[IBIS Ver]   4.2
[File Name]  stm32f2_lqfp144.ibs
[File Rev]   1.0
[Date]   31-Aug-2011
[Source]   STMicroelectronics NV
[Notes]   The I/O models have been made by simulation and qualified
   with recomandation of QualityIBIS flow.
   Some Models, library and pin names may be modified.
   Details of modified names can be found below.
ORIGINAL NAME   ::  MODIFIED NAME   :: COMMENTS(if any)
IO8USB_LSFS_OTG_FT  ::  IO8USB_LSFS_OTG_FT_USB   :: Model in USB mode.
IO8USB_LSFS_OTG_FT  ::  IO8USB_LSFS_OTG_FT_NON_USB_DNV33  :: Model in other than USB mode & pad pin = DNV33
IO8USB_LSFS_OTG_FT  ::  IO8USB_LSFS_OTG_FT_NON_USB_DPV33  :: Model in other than USB mode & pad pin = DPV33
[Disclaimer] These IBIS models are the proprietary information of
   STMicroelectronics and are disclosed to users solely for
   modeling and simulation purposes. No further license is
   implied. All warranties express, implied, or statutory,
   including any implied warranty of fitness for a particular
   purpose or implied warranty against infringement, are
   hereby disclaimed. STMicroelectronics reserves the right
   to change the IBIS models at any time and without notice.
[Copyright]  (c) STMicroelectronics
   All rights reserved. Reproduction in whole or part is prohibited
   without the written consent of the copyright holder.
[Component]  STM32F2_LQFP144
[Manufacturer] STMicroelectronics NV
[Package]
| variable   typ   min   max
R_pkg   0.000mOhm   0.000mOhm   0.000mOhm
L_pkg   0.000nH   0.000nH   0.000nH
C_pkg   0.000pF   0.000pF   0.000pF
[Pin]   signal_name   model_name
1 PE2 IO8PROG2M25M50M100M_ARSUDQ_FT
2 PE3 IO8PROG2M25M50M100M_ARSUDQ_FT
3 PE4 IO8PROG2M25M50M100M_ARSUDQ_FT
4 PE5 IO8PROG2M25M50M100M_ARSUDQ_FT
5 PE6 IO8PROG2M25M50M100M_ARSUDQ_FT
|6 VBAT VDD33IOSWCO_MOSSWI_FT
|- PI8 IO8PROG2M25M50M100M_ARSUDQ_FT_V33
7 PC13 IO8PROG2M25M50M100M_ARWSUDQ_FT_V33
8 PC14 IO8PROG2M25M50M100M_ARWSUDQ_FT
9 PC15 IO8PROG2M25M50M100M_ARSUDQ_FT
|- PI9  IO8PROG2M25M50M100M_ARSUDQ_FT
|- PI10 IO8PROG2M25M50M100M_ARSUDQ_FT
|- PI11 IO8PROG2M25M50M100M_ARSUDQ_FT
|- VSS_13 VSSIOCO
|- VDD_13 VDD33IOCO
10 PF0 IO8PROG2M25M50M100M_ARSUDQ_FT
11 PF1 IO8PROG2M25M50M100M_ARSUDQ_FT
12 PF2 IO8PROG2M25M50M100M_ARSUDQ_FT
13 PF3 IO8PROG2M25M50M100M_ARSUDQ_FT
14 PF4 IO8PROG2M25M50M100M_ARSUDQ_FT
15 PF5 IO8PROG2M25M50M100M_ARSUDQ_FT
|16 VSS_5 VSSIOCO
|17 VDD_5 VDD33IOCO
18 PF6 IO8PROG2M25M50M100M_ARSUDQ_FT
19 PF7 IO8PROG2M25M50M100M_ARSUDQ_FT
20 PF8 IO8PROG2M25M50M100M_ARSUDQ_FT
21 PF9  IO8PROG2M25M50M100M_AR3WSUDQ_FT
22 PF10 IO8PROG2M25M50M100M_ARSUDQ_FT
23 PH0 IO8PROG2M25M50M100M_ARSUDQ_FT
24 PH1 IO8PROG2M25M50M100M_ARSUDQ_FT
|25 NRST RESET
26 PC0 IO8PROG2M25M50M100M_AR3WSUDQ_FT
27 PC1 IO8PROG2M25M50M100M_AR3WSUDQ_FT
28 PC2 IO8PROG2M25M50M100M_AR3WSUDQ_FT
29 PC3 IO8PROG2M25M50M100M_AR3WSUDQ_FT
|30 VDD_12 VDD33IOCO_VSSIOCO_MOSSWI_FT
|31 VSSA VSSCO
|32 VREF+ VDD33CO
|33 VDDA VDD33CO
34 PA0 IO8PROG2M25M50M100M_AR3WSUDQ_FT_V33
35 PA1 IO8PROG2M25M50M100M_AR3WSUDQ_FT
36 PA2 IO8PROG2M25M50M100M_AR3WSUDQ_FT
|- PH2 IO8PROG2M25M50M100M_AR3WSUDQ_FT
|- PH3 IO8PROG2M25M50M100M_AR3WSUDQ_FT
|- PH4 IO8PROG2M25M50M100M_AR3WSUDQ_FT
|- PH5 IO8PROG2M25M50M100M_AR3WSUDQ_FT
37 PA3 IO8PROG2M25M50M100M_AR3WSUDQ_FT
|38 VSS_4 VSSIOCO
|39 VDD_4 VDD33IOCO
40 PA4 IO8PROG2M25M50M100M_AR3WSUDQ_FT
41 PA5 IO8PROG2M25M50M100M_AR3WSUDQ_FT
42 PA6 IO8PROG2M25M50M100M_AR3WSUDQ_FT
43 PA7 IO8PROG2M25M50M100M_AR3WSUDQ_FT
44 PC4 IO8PROG2M25M50M100M_AR3WSUDQ_FT
45 PC5 IO8PROG2M25M50M100M_AR3WSUDQ_FT
46 PB0 IO8PROG2M25M50M100M_AR3WSUDQ_FT
47 PB1 IO8PROG2M25M50M100M_AR3WSUDQ_FT
48 PB2 IO8PROG2M25M50M100M_AR3WSUDQ_FT
49 PF11 IO8PROG2M25M50M100M_ARSUDQ_FT
50 PF12 IO8PROG2M25M50M100M_ARSUDQ_FT
|51 VSS_6 VSSIOCO
|52 VDD_6 VDD33IOCO
53 PF13 IO8PROG2M25M50M100M_ARSUDQ_FT
54 PF14 IO8PROG2M25M50M100M_ARSUDQ_FT
55 PF15 IO8PROG2M25M50M100M_ARSUDQ_FT
56 PG0 IO8PROG2M25M50M100M_ARSUDQ_FT
57 PG1 IO8PROG2M25M50M100M_ARSUDQ_FT
58 PE7 IO8PROG2M25M50M100M_ARSUDQ_FT
59 PE8 IO8PROG2M25M50M100M_ARSUDQ_FT
60 PE9 IO8PROG2M25M50M100M_ARSUDQ_FT
|61 VSS_7 VSSIOCO
|62 VDD_7 VDD33IOCO
63 PE10 IO8PROG2M25M50M100M_ARSUDQ_FT
64 PE11 IO8PROG2M25M50M100M_ARSUDQ_FT
65 PE12 IO8PROG2M25M50M100M_ARSUDQ_FT
66 PE13 IO8PROG2M25M50M100M_ARSUDQ_FT
67 PE14 IO8PROG2M25M50M100M_ARSUDQ_FT
68 PE15 IO8PROG2M25M50M100M_ARSUDQ_FT
69 PB10 IO8PROG2M25M50M100M_ARSUDQ_I2CIN_FT
70 PB11 IO8PROG2M25M50M100M_ARSUDQ_I2CIN_FT
|71 VCAP_1
|72 VDD_1 VDD33IOCO
|- PH6 IO8PROG2M25M50M100M_ARSUDQ_FT
|- PH7 IO8PROG2M25M50M100M_ARSUDQ_FT
|- PH8 IO8PROG2M25M50M100M_ARSUDQ_FT
|- PH9 IO8PROG2M25M50M100M_ARSUDQ_FT
|- PH10 IO8PROG2M25M50M100M_ARSUDQ_FT
|- PH11 IO8PROG2M25M50M100M_ARSUDQ_FT
|- PH12 IO8PROG2M25M50M100M_ARSUDQ_FT
|- VSS_14 VSSIOCO
|- VDD_14 VDD33IOCO
73 PB12 IO8USB_ID_OTG_FT
74 PB13 IO8USB_VBUS_OTG_FT
75 PB14 IO8USB_LSFS_OTG_FT_USB
|75 PB14 IO8USB_LSFS_OTG_FT_NON_USB_DNV33
76 PB15 IO8USB_LSFS_OTG_FT_USB
|76 PB15 IO8USB_LSFS_OTG_FT_NON_USB_DPV3394
77 PD8 IO8PROG2M25M50M100M_ARSUDQ_FT
78 PD9 IO8PROG2M25M50M100M_ARSUDQ_FT
79 PD10 IO8PROG2M25M50M100M_ARSUDQ_FT
80 PD11 IO8PROG2M25M50M100M_ARSUDQ_FT
81 PD12 IO8PROG2M25M50M100M_ARSUDQ_FT
82 PD13 IO8PROG2M25M50M100M_ARSUDQ_FT
|83 VSS_8 VSSIOCO
|84 VDD_8 VDD33IOCO
85 PD14 IO8PROG2M25M50M100M_ARSUDQ_FT
86 PD15 IO8PROG2M25M50M100M_ARSUDQ_FT
87 PG2 IO8PROG2M25M50M100M_ARSUDQ_FT
88 PG3 IO8PROG2M25M50M100M_ARSUDQ_FT
89 PG4 IO8PROG2M25M50M100M_ARSUDQ_FT
90 PG5 IO8PROG2M25M50M100M_ARSUDQ_FT
91 PG6 IO8PROG2M25M50M100M_ARSUDQ_FT
92 PG7 IO8PROG2M25M50M100M_ARSUDQ_FT
93 PG8 IO8PROG2M25M50M100M_ARSUDQ_FT
|94 VSS_9 VSSIOCO
|95 VDD_9 VDD33IOCO
96 PC6 IO8PROG2M25M50M100M_ARSUDQ_FT
97 PC7 IO8PROG2M25M50M100M_ARSUDQ_FT
98 PC8 IO8PROG2M25M50M100M_ARSUDQ_FT
99 PC9 IO8PROG2M25M50M100M_ARSUDQ_I2CIN_FT
100 PA8 IO8PROG2M25M50M100M_ARSUDQ_I2CIN_FT
101 PA9 IO8USB_VBUS_OTG_FT
102 PA10 IO8USB_ID_OTG_FT
|103 PA11 IO8USB_LSFS_OTG_FT_USB
103 PA11 IO8USB_LSFS_OTG_FT_NON_USB_DNV33
|104 PA12 IO8USB_LSFS_OTG_FT_USB
104 PA12 IO8USB_LSFS_OTG_FT_NON_USB_DPV33
105 PA13 IO8PROG2M25M50M100M_ARSUDQ_FT
|106 VCAP_2
|107 VSS_2 VSSIOCO
|108 VDD_2 VDD33IOCO
|- PH13 IO8PROG2M25M50M100M_ARSUDQ_FT
|- PH14 IO8PROG2M25M50M100M_ARSUDQ_FT
|- PH15 IO8PROG2M25M50M100M_ARSUDQ_FT
|- PI0 IO8PROG2M25M50M100M_ARSUDQ_FT
|- PI1 IO8PROG2M25M50M100M_ARSUDQ_FT
|- PI2 IO8PROG2M25M50M100M_ARSUDQ_FT
|- PI3 IO8PROG2M25M50M100M_ARSUDQ_FT
|- VSS_15 VSSIOCO
|- VDD_15 VDD33IOCO
109 PA14 IO8PROG2M25M50M100M_ARSUDQ_FT
110 PA15 IO8PROG2M25M50M100M_AR3WSUDQ_FT
111 PC10 IO8PROG2M25M50M100M_ARSUDQ_FT
112 PC11 IO8PROG2M25M50M100M_ARSUDQ_FT
113 PC12 IO8PROG2M25M50M100M_ARSUDQ_FT
114 PD0 IO8PROG2M25M50M100M_ARSUDQ_FT
115 PD1 IO8PROG2M25M50M100M_ARSUDQ_FT
116 PD2 IO8PROG2M25M50M100M_ARSUDQ_FT
117 PD3 IO8PROG2M25M50M100M_ARSUDQ_FT
118 PD4 IO8PROG2M25M50M100M_ARSUDQ_FT
119 PD5 IO8PROG2M25M50M100M_ARSUDQ_FT
|120 VSS_10 VSSIOCO
|121 VDD_10 VDD33IOCO
122 PD6 IO8PROG2M25M50M100M_ARSUDQ_FT
123 PD7 IO8PROG2M25M50M100M_ARSUDQ_FT
124 PG9 IO8PROG2M25M50M100M_ARSUDQ_FT
125 PG10 IO8PROG2M25M50M100M_ARSUDQ_FT
126 PG11 IO8PROG2M25M50M100M_ARSUDQ_FT
127 PG12 IO8PROG2M25M50M100M_ARSUDQ_FT
128 PG13 IO8PROG2M25M50M100M_ARSUDQ_FT
129 PG14 IO8PROG2M25M50M100M_ARSUDQ_FT
|130 VSS_11 VSSIOCO
|131 VDD_11 VDD33IOCO
132 PG15 IO8PROG2M25M50M100M_ARSUDQ_FT
133 PB3 IO8PROG2M25M50M100M_ARSUDQ_FT
134 PB4 IO8PROG2M25M50M100M_ARSUDQ_FT
135 PB5 IO8PROG2M25M50M100M_AR3WSUDQ_FT
136 PB6 IO8PROG2M25M50M100M_ARSUDQ_I2CIN_FT
137 PB7 IO8PROG2M25M50M100M_ARSUDQ_I2CIN_FT
138 BOOT0 VPP_TEST_HV
139 PB8 IO8PROG2M25M50M100M_ARSUDQ_I2CIN_FT
140 PB9 IO8PROG2M25M50M100M_ARSUDQ_I2CIN_FT
141 PE0 IO8PROG2M25M50M100M_ARSUDQ_FT
142 PE1 IO8PROG2M25M50M100M_ARSUDQ_FT
|- VSS VSSIOCO
|143 RFU VSSIOCO
|144 VDD_3 VDD33IOCO
|- PI4 IO8PROG2M25M50M100M_ARSUDQ_FT
|- PI5 IO8PROG2M25M50M100M_ARSUDQ_FT
|- PI6 IO8PROG2M25M50M100M_ARSUDQ_FT
|- PI7 IO8PROG2M25M50M100M_ARSUDQ_FT
[Diff Pin]  inv_pin   vdiff tdelay_typ tdelay_min tdelay_max
75 76 200mV 0  0 0
103 104 200mV 0  0 0
[Model Selector] IO8PROG2M25M50M100M_AR3WSUDQ_FT_V33
IO8PROG2M25M50M100M_AR3WSUDQ_DRV_V33_00   DRIVER MODEL  : SPEEDAV33=0 SPEEDBV33=0
IO8PROG2M25M50M100M_AR3WSUDQ_DRV_V33_01   DRIVER MODEL  : SPEEDAV33=0 SPEEDBV33=1
IO8PROG2M25M50M100M_AR3WSUDQ_DRV_V33_10   DRIVER MODEL  : SPEEDAV33=1 SPEEDBV33=0
IO8PROG2M25M50M100M_AR3WSUDQ_DRV_V33_11   DRIVER MODEL  : SPEEDAV33=1 SPEEDBV33=1
IO8PROG2M25M50M100M_AR3WSUDQ_RCV_V33_0   CMOS RECIEVER : ENHYSV33=0  OUTPUT=ZIV33
IO8PROG2M25M50M100M_AR3WSUDQ_RCV_V33_0_T  TTL  RECIEVER : ENHYSV33=0  OUTPUT=ZIV33
IO8PROG2M25M50M100M_AR3WSUDQ_RCV_V33_1   CMOS RECIEVER : ENHYSV33=1  OUTPUT=ZIV33
IO8PROG2M25M50M100M_AR3WSUDQ_RCV_V33_1_T  TTL  RECIEVER : ENHYSV33=1  OUTPUT=ZIV33
[Model Selector] IO8PROG2M25M50M100M_AR3WSUDQ_FT
IO8PROG2M25M50M100M_AR3WSUDQ_FT_DRV_00   DRIVER MODEL  : SPEEDAV12=0 SPEEDBV12=0
IO8PROG2M25M50M100M_AR3WSUDQ_FT_DRV_01   DRIVER MODEL  : SPEEDAV12=0 SPEEDBV12=1
IO8PROG2M25M50M100M_AR3WSUDQ_FT_DRV_10   DRIVER MODEL  : SPEEDAV12=1 SPEEDBV12=0
IO8PROG2M25M50M100M_AR3WSUDQ_FT_DRV_11   DRIVER MODEL  : SPEEDAV12=1 SPEEDBV12=1
IO8PROG2M25M50M100M_AR3WSUDQ_FT_RCV_00   CMOS RECIEVER : ENHYSV12=0  OUTPUT=ZIV12
IO8PROG2M25M50M100M_AR3WSUDQ_FT_RCV_00_T  TTL  RECIEVER : ENHYSV12=0  OUTPUT=ZIV12
IO8PROG2M25M50M100M_AR3WSUDQ_FT_RCV_01   CMOS RECIEVER : ENHYSV12=0  OUTPUT=ZIV33
IO8PROG2M25M50M100M_AR3WSUDQ_FT_RCV_01_T  TTL  RECIEVER : ENHYSV12=0  OUTPUT=ZIV33
IO8PROG2M25M50M100M_AR3WSUDQ_FT_RCV_10   CMOS RECIEVER : ENHYSV12=1  OUTPUT=ZIV12
IO8PROG2M25M50M100M_AR3WSUDQ_FT_RCV_10_T  TTL  RECIEVER : ENHYSV12=1  OUTPUT=ZIV12
IO8PROG2M25M50M100M_AR3WSUDQ_FT_RCV_11   CMOS RECIEVER : ENHYSV12=1  OUTPUT=ZIV33
IO8PROG2M25M50M100M_AR3WSUDQ_FT_RCV_11_T  TTL  RECIEVER : ENHYSV12=1  OUTPUT=ZIV33
[Model Selector] IO8PROG2M25M50M100M_ARSUDQ_FT
IO8PROG2M25M50M100M_ARSUDQ_FT_DRV_00   DRIVER MODEL  : SPEEDAV12=0 SPEEDBV12=0
IO8PROG2M25M50M100M_ARSUDQ_FT_DRV_01   DRIVER MODEL  : SPEEDAV12=0 SPEEDBV12=1
IO8PROG2M25M50M100M_ARSUDQ_FT_DRV_10   DRIVER MODEL  : SPEEDAV12=1 SPEEDBV12=0
IO8PROG2M25M50M100M_ARSUDQ_FT_DRV_11   DRIVER MODEL  : SPEEDAV12=1 SPEEDBV12=1
IO8PROG2M25M50M100M_ARSUDQ_FT_RCV_00   CMOS RECIEVER : ENHYSV12=0  OUTPUT=ZIV12
IO8PROG2M25M50M100M_ARSUDQ_FT_RCV_00_T   TTL  RECIEVER : ENHYSV12=0  OUTPUT=ZIV12
IO8PROG2M25M50M100M_ARSUDQ_FT_RCV_01   CMOS RECIEVER : ENHYSV12=0  OUTPUT=ZIV33
IO8PROG2M25M50M100M_ARSUDQ_FT_RCV_01_T   TTL  RECIEVER : ENHYSV12=0  OUTPUT=ZIV33
IO8PROG2M25M50M100M_ARSUDQ_FT_RCV_10   CMOS RECIEVER : ENHYSV12=1  OUTPUT=ZIV12
IO8PROG2M25M50M100M_ARSUDQ_FT_RCV_10_T   TTL  RECIEVER : ENHYSV12=1  OUTPUT=ZIV12
IO8PROG2M25M50M100M_ARSUDQ_FT_RCV_11   CMOS RECIEVER : ENHYSV12=1  OUTPUT=ZIV33
IO8PROG2M25M50M100M_ARSUDQ_FT_RCV_11_T   TTL  RECIEVER : ENHYSV12=1  OUTPUT=ZIV33
[Model Selector] IO8PROG2M25M50M100M_ARSUDQ_I2CIN_FT
IO8PROG2M25M50M100M_ARSUDQ_I2CIN_DRV_00   DRIVER MODEL  : SPEEDAV12=0 SPEEDBV12=0
IO8PROG2M25M50M100M_ARSUDQ_I2CIN_DRV_01   DRIVER MODEL  : SPEEDAV12=0 SPEEDBV12=1
IO8PROG2M25M50M100M_ARSUDQ_I2CIN_DRV_10   DRIVER MODEL  : SPEEDAV12=1 SPEEDBV12=0
IO8PROG2M25M50M100M_ARSUDQ_I2CIN_DRV_11   DRIVER MODEL  : SPEEDAV12=1 SPEEDBV12=1
IO8PROG2M25M50M100M_I2CIN_RCV_ZII2C_00   CMOS RECIEVER : TESTI2CV12=0  HSFSV12=0
IO8PROG2M25M50M100M_I2CIN_RCV_ZII2C_00_T   TTL  RECIEVER : TESTI2CV12=0  HSFSV12=0
IO8PROG2M25M50M100M_I2CIN_RCV_ZII2C_01   CMOS RECIEVER : TESTI2CV12=0  HSFSV12=1
IO8PROG2M25M50M100M_I2CIN_RCV_ZII2C_01_T   TTL  RECIEVER : TESTI2CV12=0  HSFSV12=1
IO8PROG2M25M50M100M_I2CIN_RCV_ZII2C_10   CMOS RECIEVER : TESTI2CV12=1  HSFSV12=0
IO8PROG2M25M50M100M_I2CIN_RCV_ZII2C_10_T   TTL  RECIEVER : TESTI2CV12=1  HSFSV12=0
IO8PROG2M25M50M100M_I2CIN_RCV_ZII2C_11   CMOS RECIEVER : TESTI2CV12=1  HSFSV12=1
IO8PROG2M25M50M100M_I2CIN_RCV_ZII2C_11_T   TTL  RECIEVER : TESTI2CV12=1  HSFSV12=1
IO8PROG2M25M50M100M_I2CIN_RCV_ZIV12_0   CMOS RECIEVER : ENHYSV12=0  OUTPUT=ZIV12
IO8PROG2M25M50M100M_I2CIN_RCV_ZIV12_0_T   TTL  RECIEVER : ENHYSV12=0  OUTPUT=ZIV12
IO8PROG2M25M50M100M_I2CIN_RCV_ZIV12_1   CMOS RECIEVER : ENHYSV12=1  OUTPUT=ZIV12
IO8PROG2M25M50M100M_I2CIN_RCV_ZIV12_1_T   TTL  RECIEVER : ENHYSV12=1  OUTPUT=ZIV12
IO8PROG2M25M50M100M_I2CIN_RCV_ZIV33_0   CMOS RECIEVER : ENHYSV12=0  OUTPUT=ZIV33
IO8PROG2M25M50M100M_I2CIN_RCV_ZIV33_0_T   TTL  RECIEVER : ENHYSV12=0  OUTPUT=ZIV33
IO8PROG2M25M50M100M_I2CIN_RCV_ZIV33_1   CMOS RECIEVER : ENHYSV12=1  OUTPUT=ZIV33
IO8PROG2M25M50M100M_I2CIN_RCV_ZIV33_1_T   TTL  RECIEVER : ENHYSV12=1  OUTPUT=ZIV33
[Model Selector] IO8PROG2M25M50M100M_ARWSUDQ_FT_V33
IO8PROG2M25M50M100M_ARWSUDQ_DRV_V33_00   DRIVER MODEL  : SPEEDAV33=0 SPEEDBV33=0
IO8PROG2M25M50M100M_ARWSUDQ_DRV_V33_01   DRIVER MODEL  : SPEEDAV33=0 SPEEDBV33=1
IO8PROG2M25M50M100M_ARWSUDQ_DRV_V33_10   DRIVER MODEL  : SPEEDAV33=1 SPEEDBV33=0
IO8PROG2M25M50M100M_ARWSUDQ_DRV_V33_11   DRIVER MODEL  : SPEEDAV33=1 SPEEDBV33=1
IO8PROG2M25M50M100M_ARWSUDQ_RCV_V33_0   CMOS RECIEVER : ENHYSV33=0  OUTPUT=ZIV33
IO8PROG2M25M50M100M_ARWSUDQ_RCV_V33_0_T   TTL  RECIEVER : ENHYSV33=0  OUTPUT=ZIV33
IO8PROG2M25M50M100M_ARWSUDQ_RCV_V33_1   CMOS RECIEVER : ENHYSV33=1  OUTPUT=ZIV33
IO8PROG2M25M50M100M_ARWSUDQ_RCV_V33_1_T   TTL  RECIEVER : ENHYSV33=1  OUTPUT=ZIV33
[Model Selector] IO8PROG2M25M50M100M_ARWSUDQ_FT
IO8PROG2M25M50M100M_ARWSUDQ_FT_DRV_00   DRIVER MODEL  : SPEEDAV12=0 SPEEDBV12=0
IO8PROG2M25M50M100M_ARWSUDQ_FT_DRV_01   DRIVER MODEL  : SPEEDAV12=0 SPEEDBV12=1
IO8PROG2M25M50M100M_ARWSUDQ_FT_DRV_10   DRIVER MODEL  : SPEEDAV12=1 SPEEDBV12=0
IO8PROG2M25M50M100M_ARWSUDQ_FT_DRV_11   DRIVER MODEL  : SPEEDAV12=1 SPEEDBV12=1
IO8PROG2M25M50M100M_ARWSUDQ_FT_RCV_00   CMOS RECIEVER : ENHYSV12=0  OUTPUT=ZIV12
IO8PROG2M25M50M100M_ARWSUDQ_FT_RCV_00_T   TTL  RECIEVER : ENHYSV12=0  OUTPUT=ZIV12
IO8PROG2M25M50M100M_ARWSUDQ_FT_RCV_01   CMOS RECIEVER : ENHYSV12=0  OUTPUT=ZIV33
IO8PROG2M25M50M100M_ARWSUDQ_FT_RCV_01_T   TTL  RECIEVER : ENHYSV12=0  OUTPUT=ZIV33
IO8PROG2M25M50M100M_ARWSUDQ_FT_RCV_10   CMOS RECIEVER : ENHYSV12=1  OUTPUT=ZIV12
IO8PROG2M25M50M100M_ARWSUDQ_FT_RCV_10_T   TTL  RECIEVER : ENHYSV12=1  OUTPUT=ZIV12
IO8PROG2M25M50M100M_ARWSUDQ_FT_RCV_11   CMOS RECIEVER : ENHYSV12=1  OUTPUT=ZIV33
IO8PROG2M25M50M100M_ARWSUDQ_FT_RCV_11_T   TTL  RECIEVER : ENHYSV12=1  OUTPUT=ZIV33
[Model Selector] IO8USB_ID_OTG_FT
IO8USB_ID_OTG_FT_DRV_00   DRIVER MODEL  : SPEEDAV12=0 SPEEDBV12=0
IO8USB_ID_OTG_FT_DRV_01   DRIVER MODEL  : SPEEDAV12=0 SPEEDBV12=1
IO8USB_ID_OTG_FT_DRV_10   DRIVER MODEL  : SPEEDAV12=1 SPEEDBV12=0
IO8USB_ID_OTG_FT_DRV_11   DRIVER MODEL  : SPEEDAV12=1 SPEEDBV12=1
IO8USB_ID_OTG_FT_RCV_00   CMOS RECIEVER : ENHYSV12=0  OUTPUT=ZIV12
IO8USB_ID_OTG_FT_RCV_00_T   TTL  RECIEVER : ENHYSV12=0  OUTPUT=ZIV12
IO8USB_ID_OTG_FT_RCV_01   CMOS RECIEVER : ENHYSV12=0  OUTPUT=ZIV33
IO8USB_ID_OTG_FT_RCV_01_T   TTL  RECIEVER : ENHYSV12=0  OUTPUT=ZIV33
IO8USB_ID_OTG_FT_RCV_10   CMOS RECIEVER : ENHYSV12=1  OUTPUT=ZIV12
IO8USB_ID_OTG_FT_RCV_10_T   TTL  RECIEVER : ENHYSV12=1  OUTPUT=ZIV12
IO8USB_ID_OTG_FT_RCV_11   CMOS RECIEVER : ENHYSV12=1  OUTPUT=ZIV33
IO8USB_ID_OTG_FT_RCV_11_T   TTL  RECIEVER : ENHYSV12=1  OUTPUT=ZIV33
[Model Selector] IO8USB_LSFS_OTG_FT_USB
IO8USB_LSFS_OTG_FT_DRV_USB_0   DRIVER : USBLSFSV12=0 ENUSBV12=0
IO8USB_LSFS_OTG_FT_DRV_USB_1   DRIVER : USBLSFSV12=1 ENUSBV12=0
IO8USB_LSFS_OTG_FT_RCV_USB   USB  RECIEVER : ENHYSV12=1  OUTPUT=USBZIV12
[Model Selector] IO8USB_LSFS_OTG_FT_NON_USB_DNV33
IO8USB_LSFS_OTG_FT_DRV_IO8_DNV33_00   DRIVER : SPEEDAV12=0 SPEEDBV12=0 ENUSBV12=1
IO8USB_LSFS_OTG_FT_DRV_IO8_DNV33_01   DRIVER : SPEEDAV12=0 SPEEDBV12=1 ENUSBV12=1
IO8USB_LSFS_OTG_FT_DRV_IO8_DNV33_10   DRIVER : SPEEDAV12=1 SPEEDBV12=0 ENUSBV12=1
IO8USB_LSFS_OTG_FT_DRV_IO8_DNV33_11   DRIVER : SPEEDAV12=1 SPEEDBV12=1 ENUSBV12=1
IO8USB_LSFS_OTG_FT_RCV_IO8_ZINV12_0   CMOS RECIEVER : ENHYSV12=0  OUTPUT=ZIV12
IO8USB_LSFS_OTG_FT_RCV_IO8_ZINV12_0_T  TTL  RECIEVER : ENHYSV12=0  OUTPUT=ZIV12
IO8USB_LSFS_OTG_FT_RCV_IO8_ZINV12_1   CMOS RECIEVER : ENHYSV12=1  OUTPUT=ZIV12
IO8USB_LSFS_OTG_FT_RCV_IO8_ZINV12_1_T  TTL  RECIEVER : ENHYSV12=1  OUTPUT=ZIV12
IO8USB_LSFS_OTG_FT_RCV_IO8_ZINV33_0   CMOS RECIEVER : ENHYSV12=0  OUTPUT=ZIV33
IO8USB_LSFS_OTG_FT_RCV_IO8_ZINV33_0_T  TTL  RECIEVER : ENHYSV12=0  OUTPUT=ZIV33
IO8USB_LSFS_OTG_FT_RCV_IO8_ZINV33_1   CMOS RECIEVER : ENHYSV12=1  OUTPUT=ZIV33
IO8USB_LSFS_OTG_FT_RCV_IO8_ZINV33_1_T  TTL  RECIEVER : ENHYSV12=1  OUTPUT=ZIV33
[Model Selector] IO8USB_LSFS_OTG_FT_NON_USB_DPV33
IO8USB_LSFS_OTG_FT_DRV_IO8_DPV33_00   DRIVER : SPEEDAV12=0 SPEEDBV12=0 ENUSBV12=1
IO8USB_LSFS_OTG_FT_DRV_IO8_DPV33_01   DRIVER : SPEEDAV12=0 SPEEDBV12=1 ENUSBV12=1
IO8USB_LSFS_OTG_FT_DRV_IO8_DPV33_10   DRIVER : SPEEDAV12=1 SPEEDBV12=0 ENUSBV12=1
IO8USB_LSFS_OTG_FT_DRV_IO8_DPV33_11   DRIVER : SPEEDAV12=1 SPEEDBV12=1 ENUSBV12=1
IO8USB_LSFS_OTG_FT_RCV_IO8_ZIPV12_0   CMOS RECIEVER : ENHYSV12=0  OUTPUT=ZIV12
IO8USB_LSFS_OTG_FT_RCV_IO8_ZIPV12_0_T  TTL  RECIEVER : ENHYSV12=0  OUTPUT=ZIV12
IO8USB_LSFS_OTG_FT_RCV_IO8_ZIPV12_1   CMOS RECIEVER : ENHYSV12=1  OUTPUT=ZIV12
IO8USB_LSFS_OTG_FT_RCV_IO8_ZIPV12_1_T  TTL  RECIEVER : ENHYSV12=1  OUTPUT=ZIV12
IO8USB_LSFS_OTG_FT_RCV_IO8_ZIPV33_0   CMOS RECIEVER : ENHYSV12=0  OUTPUT=ZIV33
IO8USB_LSFS_OTG_FT_RCV_IO8_ZIPV33_0_T  TTL  RECIEVER : ENHYSV12=0  OUTPUT=ZIV33
IO8USB_LSFS_OTG_FT_RCV_IO8_ZIPV33_1   CMOS RECIEVER : ENHYSV12=1  OUTPUT=ZIV33
IO8USB_LSFS_OTG_FT_RCV_IO8_ZIPV33_1_T  TTL  RECIEVER : ENHYSV12=1  OUTPUT=ZIV33
[Model Selector] IO8USB_VBUS_OTG_FT
IO8USB_VBUS_OTG_FT_DRV_00   DRIVER MODEL  : SPEEDAV12=0 SPEEDBV12=0
IO8USB_VBUS_OTG_FT_DRV_01   DRIVER MODEL  : SPEEDAV12=0 SPEEDBV12=1
IO8USB_VBUS_OTG_FT_DRV_10   DRIVER MODEL  : SPEEDAV12=1 SPEEDBV12=0
IO8USB_VBUS_OTG_FT_DRV_11   DRIVER MODEL  : SPEEDAV12=1 SPEEDBV12=1
IO8USB_VBUS_OTG_FT_RCV_00   CMOS RECIEVER : ENHYSV12=0  OUTPUT=ZIV12
IO8USB_VBUS_OTG_FT_RCV_00_T   TTL  RECIEVER : ENHYSV12=0  OUTPUT=ZIV12
IO8USB_VBUS_OTG_FT_RCV_01   CMOS RECIEVER : ENHYSV12=0  OUTPUT=ZIV33
IO8USB_VBUS_OTG_FT_RCV_01_T   TTL  RECIEVER : ENHYSV12=0  OUTPUT=ZIV33
IO8USB_VBUS_OTG_FT_RCV_10   CMOS RECIEVER : ENHYSV12=1  OUTPUT=ZIV12
IO8USB_VBUS_OTG_FT_RCV_10_T   TTL  RECIEVER : ENHYSV12=1  OUTPUT=ZIV12
IO8USB_VBUS_OTG_FT_RCV_11   CMOS RECIEVER : ENHYSV12=1  OUTPUT=ZIV33
IO8USB_VBUS_OTG_FT_RCV_11_T   TTL  RECIEVER : ENHYSV12=1  OUTPUT=ZIV33
[Model Selector] VPP_TEST_HV
VPP_TEST_HV_00   CMOS RECIEVER : ENHYSV12=0  OUTPUT=ZIV12
VPP_TEST_HV_00_T   TTL  RECIEVER : ENHYSV12=0  OUTPUT=ZIV12
VPP_TEST_HV_01   CMOS RECIEVER : ENHYSV12=0  OUTPUT=ZIV33
VPP_TEST_HV_01_T   TTL  RECIEVER : ENHYSV12=0  OUTPUT=ZIV33
VPP_TEST_HV_10   CMOS RECIEVER : ENHYSV12=1  OUTPUT=ZIV12
VPP_TEST_HV_10_T   TTL  RECIEVER : ENHYSV12=1  OUTPUT=ZIV12
VPP_TEST_HV_11   CMOS RECIEVER : ENHYSV12=1  OUTPUT=ZIV33
VPP_TEST_HV_11_T   TTL  RECIEVER : ENHYSV12=1  OUTPUT=ZIV33
| Models and submodels in the file (131): IO8PROG2M25M50M100M_AR3WSUDQ_DRV_V33_00 (3-state), IO8PROG2M25M50M100M_AR3WSUDQ_DRV_V33_01 (3-state), IO8PROG2M25M50M100M_AR3WSUDQ_DRV_V33_10 (3-state), IO8PROG2M25M50M100M_AR3WSUDQ_DRV_V33_11 (3-state), IO8PROG2M25M50M100M_AR3WSUDQ_FT_DRV_00 (3-state), IO8PROG2M25M50M100M_AR3WSUDQ_FT_DRV_01 (3-state), IO8PROG2M25M50M100M_AR3WSUDQ_FT_DRV_10 (3-state), IO8PROG2M25M50M100M_AR3WSUDQ_FT_DRV_11 (3-state), IO8PROG2M25M50M100M_AR3WSUDQ_FT_RCV_00 (Input), IO8PROG2M25M50M100M_AR3WSUDQ_FT_RCV_00_T (Input), IO8PROG2M25M50M100M_AR3WSUDQ_FT_RCV_01 (Input), IO8PROG2M25M50M100M_AR3WSUDQ_FT_RCV_01_T (Input), IO8PROG2M25M50M100M_AR3WSUDQ_FT_RCV_10 (Input), IO8PROG2M25M50M100M_AR3WSUDQ_FT_RCV_10_T (Input), IO8PROG2M25M50M100M_AR3WSUDQ_FT_RCV_11 (Input), IO8PROG2M25M50M100M_AR3WSUDQ_FT_RCV_11_T (Input), IO8PROG2M25M50M100M_AR3WSUDQ_RCV_V33_0 (Input), IO8PROG2M25M50M100M_AR3WSUDQ_RCV_V33_0_T (Input), IO8PROG2M25M50M100M_AR3WSUDQ_RCV_V33_1 (Input), IO8PROG2M25M50M100M_AR3WSUDQ_RCV_V33_1_T (Input), IO8PROG2M25M50M100M_ARSUDQ_FT_DRV_00 (3-state), IO8PROG2M25M50M100M_ARSUDQ_FT_DRV_01 (3-state), IO8PROG2M25M50M100M_ARSUDQ_FT_DRV_10 (3-state), IO8PROG2M25M50M100M_ARSUDQ_FT_DRV_11 (3-state), IO8PROG2M25M50M100M_ARSUDQ_FT_RCV_00 (Input), IO8PROG2M25M50M100M_ARSUDQ_FT_RCV_00_T (Input), IO8PROG2M25M50M100M_ARSUDQ_FT_RCV_01 (Input), IO8PROG2M25M50M100M_ARSUDQ_FT_RCV_01_T (Input), IO8PROG2M25M50M100M_ARSUDQ_FT_RCV_10 (Input), IO8PROG2M25M50M100M_ARSUDQ_FT_RCV_10_T (Input), IO8PROG2M25M50M100M_ARSUDQ_FT_RCV_11 (Input), IO8PROG2M25M50M100M_ARSUDQ_FT_RCV_11_T (Input), IO8PROG2M25M50M100M_ARSUDQ_I2CIN_DRV_00 (3-state), IO8PROG2M25M50M100M_ARSUDQ_I2CIN_DRV_01 (3-state), IO8PROG2M25M50M100M_ARSUDQ_I2CIN_DRV_10 (3-state), IO8PROG2M25M50M100M_ARSUDQ_I2CIN_DRV_11 (3-state), IO8PROG2M25M50M100M_ARWSUDQ_DRV_V33_00 (3-state), IO8PROG2M25M50M100M_ARWSUDQ_DRV_V33_01 (3-state), IO8PROG2M25M50M100M_ARWSUDQ_DRV_V33_10 (3-state), IO8PROG2M25M50M100M_ARWSUDQ_DRV_V33_11 (3-state), IO8PROG2M25M50M100M_ARWSUDQ_FT_DRV_00 (3-state), IO8PROG2M25M50M100M_ARWSUDQ_FT_DRV_01 (3-state), IO8PROG2M25M50M100M_ARWSUDQ_FT_DRV_10 (3-state), IO8PROG2M25M50M100M_ARWSUDQ_FT_DRV_11 (3-state), IO8PROG2M25M50M100M_ARWSUDQ_FT_RCV_00 (Input), IO8PROG2M25M50M100M_ARWSUDQ_FT_RCV_00_T (Input), IO8PROG2M25M50M100M_ARWSUDQ_FT_RCV_01 (Input), IO8PROG2M25M50M100M_ARWSUDQ_FT_RCV_01_T (Input), IO8PROG2M25M50M100M_ARWSUDQ_FT_RCV_10 (Input), IO8PROG2M25M50M100M_ARWSUDQ_FT_RCV_10_T (Input), IO8PROG2M25M50M100M_ARWSUDQ_FT_RCV_11 (Input), IO8PROG2M25M50M100M_ARWSUDQ_FT_RCV_11_T (Input), IO8PROG2M25M50M100M_ARWSUDQ_RCV_V33_0 (Input), IO8PROG2M25M50M100M_ARWSUDQ_RCV_V33_0_T (Input), IO8PROG2M25M50M100M_ARWSUDQ_RCV_V33_1 (Input), IO8PROG2M25M50M100M_ARWSUDQ_RCV_V33_1_T (Input), IO8PROG2M25M50M100M_I2CIN_RCV_ZII2C_00 (Input), IO8PROG2M25M50M100M_I2CIN_RCV_ZII2C_00_T (Input), IO8PROG2M25M50M100M_I2CIN_RCV_ZII2C_01 (Input), IO8PROG2M25M50M100M_I2CIN_RCV_ZII2C_01_T (Input), IO8PROG2M25M50M100M_I2CIN_RCV_ZII2C_10 (Input), IO8PROG2M25M50M100M_I2CIN_RCV_ZII2C_10_T (Input), IO8PROG2M25M50M100M_I2CIN_RCV_ZII2C_11 (Input), IO8PROG2M25M50M100M_I2CIN_RCV_ZII2C_11_T (Input), IO8PROG2M25M50M100M_I2CIN_RCV_ZIV12_0 (Input), IO8PROG2M25M50M100M_I2CIN_RCV_ZIV12_0_T (Input), IO8PROG2M25M50M100M_I2CIN_RCV_ZIV12_1 (Input), IO8PROG2M25M50M100M_I2CIN_RCV_ZIV12_1_T (Input), IO8PROG2M25M50M100M_I2CIN_RCV_ZIV33_0 (Input), IO8PROG2M25M50M100M_I2CIN_RCV_ZIV33_0_T (Input), IO8PROG2M25M50M100M_I2CIN_RCV_ZIV33_1 (Input), IO8PROG2M25M50M100M_I2CIN_RCV_ZIV33_1_T (Input), IO8USB_ID_OTG_FT_DRV_00 (3-state), IO8USB_ID_OTG_FT_DRV_01 (3-state), IO8USB_ID_OTG_FT_DRV_10 (3-state), IO8USB_ID_OTG_FT_DRV_11 (3-state), IO8USB_ID_OTG_FT_RCV_00 (Input), IO8USB_ID_OTG_FT_RCV_00_T (Input), IO8USB_ID_OTG_FT_RCV_01 (Input), IO8USB_ID_OTG_FT_RCV_01_T (Input)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
